| IBIS file stm32u575_585_wlcsp90_smps.ibs
[IBIS ver] 4.2
[File name] stm32u575_585_wlcsp90_smps.ibs
[File Rev] 1.0
[Date]  06-08-2021
[Source] Data Created at STMicroelectronics
[Notes]  File originated from ELDO simulations.
[Disclaimer]  This information is for modeling purpose only and is
   not guaranted. The information is subject to change without
   notice.
[Copyright] Copyright 2021 STMicroelectronics Inc.
|   Component stm32u575_585_wlcsp90_smps
[Component] stm32u575_585_wlcsp90_smps
[Manufacturer] STMicroelectronics
[Package]
| variable   typ   min   max
R_pkg   0   NA   NA
L_pkg   0   NA   NA
C_pkg   0   NA   NA
[Pin]   signal_name   model_name   R_pin   L_pin   C_pin   | Comment
A1 VDD POWER
A11 VDDIO2 POWER
A13 PB6 io8_100m_i2c_ft
A15 PB9 io8_100m_i2c_ft
A17 VDD11 POWER
A3 PC11 io8_100m_hslv_ft
A5 PD2 io8_100m_ft
A7 PG10 io8_100m_hslv_ft
A9 PG14 io8_100m_hslv_ft
B10 VSS GND
B12 PB7 io8_166m_hslv_i2c_ft
B14 PB8 io8_100m_i2c_ft
B16 VSS GND
B18 VDD POWER
B2 VSS GND
B4 PC12 io8_166m_hslv_ft
B6 PD5 io8_100m_hslv_ft
B8 PG12 io8_100m_hslv_ft
C1 VDDUSB POWER
C11 PB4 io8_100m_i2c_ft
C13 PH3-BOOT0 io8_100m_ft
C15 PE3 io8_100m_hslv_tamp_ft
C17 VBAT POWER
C3 PA14 io8_100m_ft
C5 PD0 io8_100m_hslv_ft
C7 PG9 io8_100m_hslv_ft
C9 PG13 io8_100m_hslv_ft
D10 PB3 io8_100m_i2c_ft
D12 PB5 io8_166m_hslv_ft
D14 PE4 io8_100m_hslv_tamp_ft
D16 PE6 io8_100m_hslv_tamp_ft
D18 PC14-OSC32_IN io8_100m_ft
D2 PA12 io8_usb_ft
D4 PA13 io8_100m_ft
D6 PD1 io8_100m_hslv_ft
D8 PD4 io8_100m_hslv_ft
E1 PA10 io8_100m_usb_id
E11 PA9 io8_100m_usb_vbus_ft
E13 PE5 io8_100m_hslv_tamp_ft
E15 PC13 io8_100m_ft_v33
E17 PC15-OSC32_OUT io8_100m_ft
E3 PA11 io8_usb_ft
E5 PA15 nc
E7 PC10 io8_100m_ft
E9 PG11 io8_100m_hslv_ft
F10 PA6 io8_100m_hslv_ft
F12 PC2 io8_100m_hslv_ft
F14 PC0 io8_100m_hslv_ft
F16 PH1-OSC_OUT io8_100m_ft
F18 PH0-OSC_IN io8_100m_ft
F2 PC8 io8_100m_ft
F4 PC7 io8_100m_ft
F6 PC9 io8_100m_ft
F8 PA8 io8_166m_hslv_ft
G1 PD14 io8_100m_hslv_ft
G11 PA0 io8_100m_hslv_tamp_ft
G13 PC3 io8_100m_hslv_ft
G15 PC1 io8_166m_hslv_i2c_ft
G17 NRST nc
G3 PD15 io8_100m_hslv_ft
G5 PB15 nc
G7 PC6 io8_100m_ft
G9 PC5 io8_100m_tamp_ft
H10 PA3 io8_166m_hslv_ft
H12 PA5 io8_100m_ft
H14 PA4 io8_100m_hslv_ft
H16 VREF+ POWER
H18 VSSA GND
H2 PB13 io8_100m_i2c_ft
H4 PB14 io8_100m_i2c_ft
H6 PB10 io8_166m_hslv_i2c_ft
H8 PE7 io8_100m_hslv_ft
J1 VDD POWER
J11 PB1 io8_100m_hslv_ft
J13 PA1 io8_100m_hslv_tamp_ft
J15 PA2 io8_100m_hslv_ft
J17 VDDA POWER
J3 VSS GND
J5 VSSSMPS GND
J7 PE10 io8_166m_hslv_ft
J9 PE8 io8_100m_hslv_ft
K10 PB2 io8_100m_hslv_tamp_ft
K12 PB0 io8_100m_hslv_ft
K14 PA7 io8_100m_hslv_ft
K16 VDD POWER
K18 VSS GND
K1 VDD11 POWER
K4 VDDSMPS POWER
K6 VLXSMPS POWER
K8 PE9 io8_166m_hslv_ft
[Model Selector] io8_100m_ft
io8_100m_ft_hs_1v2  "IO8_FT 100MHz high speed @ 1.2V"
io8_100m_ft_hs_pu_1v2  "IO8_FT 100MHz high speed @ 1.2V pullup"
io8_100m_ft_hs_pd_1v2  "IO8_FT 100MHz high speed @ 1.2V pulldown"
io8_100m_ft_fs_1v2  "IO8_FT 100MHz fast speed @ 1.2V"
io8_100m_ft_fs_pu_1v2  "IO8_FT 100MHz fast speed @ 1.2V pullup"
io8_100m_ft_fs_pd_1v2  "IO8_FT 100MHz fast speed @ 1.2V pulldown"
io8_100m_ft_ms_1v2  "IO8_FT 100MHz med speed @ 1.2V"
io8_100m_ft_ms_pu_1v2  "IO8_FT 100MHz med speed @ 1.2V pullup"
io8_100m_ft_ms_pd_1v2  "IO8_FT 100MHz med speed @ 1.2V pulldown"
io8_100m_ft_ls_1v2  "IO8_FT 100MHz low speed @ 1.2V"
io8_100m_ft_ls_pu_1v2  "IO8_FT 100MHz low speed @ 1.2V pullup"
io8_100m_ft_ls_pd_1v2  "IO8_FT 100MHz low speed @ 1.2V pulldown"
io8_100m_ft_hs_1v8  "IO8_FT 100MHz high speed @ 1.8V"
io8_100m_ft_hs_pu_1v8  "IO8_FT 100MHz high speed @ 1.8V pullup"
io8_100m_ft_hs_pd_1v8  "IO8_FT 100MHz high speed @ 1.8V pulldown"
io8_100m_ft_fs_1v8  "IO8_FT 100MHz fast speed @ 1.8V"
io8_100m_ft_fs_pu_1v8  "IO8_FT 100MHz fast speed @ 1.8V pullup"
io8_100m_ft_fs_pd_1v8  "IO8_FT 100MHz fast speed @ 1.8V pulldown"
io8_100m_ft_ms_1v8  "IO8_FT 100MHz med speed @ 1.8V"
io8_100m_ft_ms_pu_1v8  "IO8_FT 100MHz med speed @ 1.8V pullup"
io8_100m_ft_ms_pd_1v8  "IO8_FT 100MHz med speed @ 1.8V pulldown"
io8_100m_ft_ls_1v8  "IO8_FT 100MHz low speed @ 1.8V"
io8_100m_ft_ls_pu_1v8  "IO8_FT 100MHz low speed @ 1.8V pullup"
io8_100m_ft_ls_pd_1v8  "IO8_FT 100MHz low speed @ 1.8V pulldown"
io8_100m_ft_hs_3v3  "IO8_FT 100MHz high speed @ 3.3V"
io8_100m_ft_hs_pu_3v3  "IO8_FT 100MHz high speed @ 3.3V pullup"
io8_100m_ft_hs_pd_3v3  "IO8_FT 100MHz high speed @ 3.3V pulldown"
io8_100m_ft_fs_3v3  "IO8_FT 100MHz fast speed @ 3.3V"
io8_100m_ft_fs_pu_3v3  "IO8_FT 100MHz fast speed @ 3.3V pullup"
io8_100m_ft_fs_pd_3v3  "IO8_FT 100MHz fast speed @ 3.3V pulldown"
io8_100m_ft_ms_3v3  "IO8_FT 100MHz med speed @ 3.3V"
io8_100m_ft_ms_pu_3v3  "IO8_FT 100MHz med speed @ 3.3V pullup"
io8_100m_ft_ms_pd_3v3  "IO8_FT 100MHz med speed @ 3.3V pulldown"
io8_100m_ft_ls_3v3  "IO8_FT 100MHz low speed @ 3.3V"
io8_100m_ft_ls_pu_3v3  "IO8_FT 100MHz low speed @ 3.3V pullup"
io8_100m_ft_ls_pd_3v3  "IO8_FT 100MHz low speed @ 3.3V pulldown"
[Model Selector] io8_100m_hslv_ft
io8_100m_ft_hs_1v2  "IO8_FT 100MHz high speed @ 1.2V"
io8_100m_ft_hs_pu_1v2  "IO8_FT 100MHz high speed @ 1.2V pullup"
io8_100m_ft_hs_pd_1v2  "IO8_FT 100MHz high speed @ 1.2V pulldown"
io8_100m_ft_fs_1v2  "IO8_FT 100MHz fast speed @ 1.2V"
io8_100m_ft_fs_pu_1v2  "IO8_FT 100MHz fast speed @ 1.2V pullup"
io8_100m_ft_fs_pd_1v2  "IO8_FT 100MHz fast speed @ 1.2V pulldown"
io8_100m_ft_ms_1v2  "IO8_FT 100MHz med speed @ 1.2V"
io8_100m_ft_ms_pu_1v2  "IO8_FT 100MHz med speed @ 1.2V pullup"
io8_100m_ft_ms_pd_1v2  "IO8_FT 100MHz med speed @ 1.2V pulldown"
io8_100m_ft_ls_1v2  "IO8_FT 100MHz low speed @ 1.2V"
io8_100m_ft_ls_pu_1v2  "IO8_FT 100MHz low speed @ 1.2V pullup"
io8_100m_ft_ls_pd_1v2  "IO8_FT 100MHz low speed @ 1.2V pulldown"
io8_100m_ft_hs_1v8  "IO8_FT 100MHz high speed @ 1.8V"
io8_100m_ft_hs_pu_1v8  "IO8_FT 100MHz high speed @ 1.8V pullup"
io8_100m_ft_hs_pd_1v8  "IO8_FT 100MHz high speed @ 1.8V pulldown"
io8_100m_ft_fs_1v8  "IO8_FT 100MHz fast speed @ 1.8V"
io8_100m_ft_fs_pu_1v8  "IO8_FT 100MHz fast speed @ 1.8V pullup"
io8_100m_ft_fs_pd_1v8  "IO8_FT 100MHz fast speed @ 1.8V pulldown"
io8_100m_ft_ms_1v8  "IO8_FT 100MHz med speed @ 1.8V"
io8_100m_ft_ms_pu_1v8  "IO8_FT 100MHz med speed @ 1.8V pullup"
io8_100m_ft_ms_pd_1v8  "IO8_FT 100MHz med speed @ 1.8V pulldown"
io8_100m_ft_ls_1v8  "IO8_FT 100MHz low speed @ 1.8V"
io8_100m_ft_ls_pu_1v8  "IO8_FT 100MHz low speed @ 1.8V pullup"
io8_100m_ft_ls_pd_1v8  "IO8_FT 100MHz low speed @ 1.8V pulldown"
io8_100m_ft_hs_3v3  "IO8_FT 100MHz high speed @ 3.3V"
io8_100m_ft_hs_pu_3v3  "IO8_FT 100MHz high speed @ 3.3V pullup"
io8_100m_ft_hs_pd_3v3  "IO8_FT 100MHz high speed @ 3.3V pulldown"
io8_100m_ft_fs_3v3  "IO8_FT 100MHz fast speed @ 3.3V"
io8_100m_ft_fs_pu_3v3  "IO8_FT 100MHz fast speed @ 3.3V pullup"
io8_100m_ft_fs_pd_3v3  "IO8_FT 100MHz fast speed @ 3.3V pulldown"
io8_100m_ft_ms_3v3  "IO8_FT 100MHz med speed @ 3.3V"
io8_100m_ft_ms_pu_3v3  "IO8_FT 100MHz med speed @ 3.3V pullup"
io8_100m_ft_ms_pd_3v3  "IO8_FT 100MHz med speed @ 3.3V pulldown"
io8_100m_ft_ls_3v3  "IO8_FT 100MHz low speed @ 3.3V"
io8_100m_ft_ls_pu_3v3  "IO8_FT 100MHz low speed @ 3.3V pullup"
io8_100m_ft_ls_pd_3v3  "IO8_FT 100MHz low speed @ 3.3V pulldown"
io8_100m_hslv_ft_hs_1v2  "IO8_FT 100MHz HSLV high speed @ 1.2V"
io8_100m_hslv_ft_hs_pu_1v2  "IO8_FT 100MHz HSLV high speed @ 1.2V pullup"
io8_100m_hslv_ft_hs_pd_1v2  "IO8_FT 100MHz HSLV high speed @ 1.2V pulldown"
io8_100m_hslv_ft_fs_1v2  "IO8_FT 100MHz HSLV fast speed @ 1.2V"
io8_100m_hslv_ft_fs_pu_1v2  "IO8_FT 100MHz HSLV fast speed @ 1.2V pullup"
io8_100m_hslv_ft_fs_pd_1v2  "IO8_FT 100MHz HSLV fast speed @ 1.2V pulldown"
io8_100m_hslv_ft_ms_1v2  "IO8_FT 100MHz HSLV med speed @ 1.2V"
io8_100m_hslv_ft_ms_pu_1v2  "IO8_FT 100MHz HSLV med speed @ 1.2V pullup"
io8_100m_hslv_ft_ms_pd_1v2  "IO8_FT 100MHz HSLV med speed @ 1.2V pulldown"
io8_100m_hslv_ft_ls_1v2  "IO8_FT 100MHz HSLV low speed @ 1.2V"
io8_100m_hslv_ft_ls_pu_1v2  "IO8_FT 100MHz HSLV low speed @ 1.2V pullup"
io8_100m_hslv_ft_ls_pd_1v2  "IO8_FT 100MHz HSLV low speed @ 1.2V pulldown"
io8_100m_hslv_ft_hs_1v8  "IO8_FT 100MHz HSLV high speed @ 1.8V"
io8_100m_hslv_ft_hs_pu_1v8  "IO8_FT 100MHz HSLV high speed @ 1.8V pullup"
io8_100m_hslv_ft_hs_pd_1v8  "IO8_FT 100MHz HSLV high speed @ 1.8V pulldown"
io8_100m_hslv_ft_fs_1v8  "IO8_FT 100MHz HSLV fast speed @ 1.8V"
io8_100m_hslv_ft_fs_pu_1v8  "IO8_FT 100MHz HSLV fast speed @ 1.8V pullup"
io8_100m_hslv_ft_fs_pd_1v8  "IO8_FT 100MHz HSLV fast speed @ 1.8V pulldown"
io8_100m_hslv_ft_ms_1v8  "IO8_FT 100MHz HSLV med speed @ 1.8V"
io8_100m_hslv_ft_ms_pu_1v8  "IO8_FT 100MHz HSLV med speed @ 1.8V pullup"
io8_100m_hslv_ft_ms_pd_1v8  "IO8_FT 100MHz HSLV med speed @ 1.8V pulldown"
io8_100m_hslv_ft_ls_1v8  "IO8_FT 100MHz HSLV low speed @ 1.8V"
io8_100m_hslv_ft_ls_pu_1v8  "IO8_FT 100MHz HSLV low speed @ 1.8V pullup"
io8_100m_hslv_ft_ls_pd_1v8  "IO8_FT 100MHz HSLV low speed @ 1.8V pulldown"
io8_100m_hslv_ft_hs_2v5  "IO8_FT 100MHz HSLV high speed @ 2.5V"
io8_100m_hslv_ft_hs_pu_2v5  "IO8_FT 100MHz HSLV high speed @ 2.5V pullup"
io8_100m_hslv_ft_hs_pd_2v5  "IO8_FT 100MHz HSLV high speed @ 2.5V pulldown"
io8_100m_hslv_ft_fs_2v5  "IO8_FT 100MHz HSLV fast speed @ 2.5V"
io8_100m_hslv_ft_fs_pu_2v5  "IO8_FT 100MHz HSLV fast speed @ 2.5V pullup"
io8_100m_hslv_ft_fs_pd_2v5  "IO8_FT 100MHz HSLV fast speed @ 2.5V pulldown"
io8_100m_hslv_ft_ms_2v5  "IO8_FT 100MHz HSLV med speed @ 2.5V"
io8_100m_hslv_ft_ms_pu_2v5  "IO8_FT 100MHz HSLV med speed @ 2.5V pullup"
io8_100m_hslv_ft_ms_pd_2v5  "IO8_FT 100MHz HSLV med speed @ 2.5V pulldown"
io8_100m_hslv_ft_ls_2v5  "IO8_FT 100MHz HSLV low speed @ 2.5V"
io8_100m_hslv_ft_ls_pu_2v5  "IO8_FT 100MHz HSLV low speed @ 2.5V pullup"
io8_100m_hslv_ft_ls_pd_2v5  "IO8_FT 100MHz HSLV low speed @ 2.5V pulldown"
[Model Selector] io8_166m_hslv_ft
io8_166m_ft_hs_1v2  "IO8_FT 166MHz high speed @ 1.2V"
io8_166m_ft_hs_pu_1v2  "IO8_FT 166MHz high speed @ 1.2V pullup"
io8_166m_ft_hs_pd_1v2  "IO8_FT 166MHz high speed @ 1.2V pulldown"
io8_166m_ft_fs_1v2  "IO8_FT 166MHz fast speed @ 1.2V"
io8_166m_ft_fs_pu_1v2  "IO8_FT 166MHz fast speed @ 1.2V pullup"
io8_166m_ft_fs_pd_1v2  "IO8_FT 166MHz fast speed @ 1.2V pulldown"
io8_166m_ft_ms_1v2  "IO8_FT 166MHz med speed @ 1.2V"
io8_166m_ft_ms_pu_1v2  "IO8_FT 166MHz med speed @ 1.2V pullup"
io8_166m_ft_ms_pd_1v2  "IO8_FT 166MHz med speed @ 1.2V pulldown"
io8_166m_ft_ls_1v2  "IO8_FT 166MHz low speed @ 1.2V"
io8_166m_ft_ls_pu_1v2  "IO8_FT 166MHz low speed @ 1.2V pullup"
io8_166m_ft_ls_pd_1v2  "IO8_FT 166MHz low speed @ 1.2V pulldown"
io8_166m_ft_hs_1v8  "IO8_FT 166MHz high speed @ 1.8V"
io8_166m_ft_hs_pu_1v8  "IO8_FT 166MHz high speed @ 1.8V pullup"
io8_166m_ft_hs_pd_1v8  "IO8_FT 166MHz high speed @ 1.8V pulldown"
io8_166m_ft_fs_1v8  "IO8_FT 166MHz fast speed @ 1.8V"
io8_166m_ft_fs_pu_1v8  "IO8_FT 166MHz fast speed @ 1.8V pullup"
io8_166m_ft_fs_pd_1v8  "IO8_FT 166MHz fast speed @ 1.8V pulldown"
io8_166m_ft_ms_1v8  "IO8_FT 166MHz med speed @ 1.8V"
io8_166m_ft_ms_pu_1v8  "IO8_FT 166MHz med speed @ 1.8V pullup"
io8_166m_ft_ms_pd_1v8  "IO8_FT 166MHz med speed @ 1.8V pulldown"
io8_166m_ft_ls_1v8  "IO8_FT 166MHz low speed @ 1.8V"
io8_166m_ft_ls_pu_1v8  "IO8_FT 166MHz low speed @ 1.8V pullup"
io8_166m_ft_ls_pd_1v8  "IO8_FT 166MHz low speed @ 1.8V pulldown"
io8_166m_ft_hs_3v3  "IO8_FT 166MHz high speed @ 3.3V"
io8_166m_ft_hs_pu_3v3  "IO8_FT 166MHz high speed @ 3.3V pullup"
io8_166m_ft_hs_pd_3v3  "IO8_FT 166MHz high speed @ 3.3V pulldown"
io8_166m_ft_fs_3v3  "IO8_FT 166MHz fast speed @ 3.3V"
io8_166m_ft_fs_pu_3v3  "IO8_FT 166MHz fast speed @ 3.3V pullup"
io8_166m_ft_fs_pd_3v3  "IO8_FT 166MHz fast speed @ 3.3V pulldown"
io8_166m_ft_ms_3v3  "IO8_FT 166MHz med speed @ 3.3V"
io8_166m_ft_ms_pu_3v3  "IO8_FT 166MHz med speed @ 3.3V pullup"
io8_166m_ft_ms_pd_3v3  "IO8_FT 166MHz med speed @ 3.3V pulldown"
io8_166m_ft_ls_3v3  "IO8_FT 166MHz low speed @ 3.3V"
io8_166m_ft_ls_pu_3v3  "IO8_FT 166MHz low speed @ 3.3V pullup"
io8_166m_ft_ls_pd_3v3  "IO8_FT 166MHz low speed @ 3.3V pulldown"
io8_166m_hslv_ft_hs_1v2  "IO8_FT 166MHz HSLV high speed @ 1.2V"
io8_166m_hslv_ft_hs_pu_1v2  "IO8_FT 166MHz HSLV high speed @ 1.2V pullup"
io8_166m_hslv_ft_hs_pd_1v2  "IO8_FT 166MHz HSLV high speed @ 1.2V pulldown"
io8_166m_hslv_ft_fs_1v2  "IO8_FT 166MHz HSLV fast speed @ 1.2V"
io8_166m_hslv_ft_fs_pu_1v2  "IO8_FT 166MHz HSLV fast speed @ 1.2V pullup"
io8_166m_hslv_ft_fs_pd_1v2  "IO8_FT 166MHz HSLV fast speed @ 1.2V pulldown"
io8_166m_hslv_ft_ms_1v2  "IO8_FT 166MHz HSLV med speed @ 1.2V"
io8_166m_hslv_ft_ms_pu_1v2  "IO8_FT 166MHz HSLV med speed @ 1.2V pullup"
io8_166m_hslv_ft_ms_pd_1v2  "IO8_FT 166MHz HSLV med speed @ 1.2V pulldown"
io8_166m_hslv_ft_ls_1v2  "IO8_FT 166MHz HSLV low speed @ 1.2V"
io8_166m_hslv_ft_ls_pu_1v2  "IO8_FT 166MHz HSLV low speed @ 1.2V pullup"
io8_166m_hslv_ft_ls_pd_1v2  "IO8_FT 166MHz HSLV low speed @ 1.2V pulldown"
io8_166m_hslv_ft_hs_1v8  "IO8_FT 166MHz HSLV high speed @ 1.8V"
io8_166m_hslv_ft_hs_pu_1v8  "IO8_FT 166MHz HSLV high speed @ 1.8V pullup"
io8_166m_hslv_ft_hs_pd_1v8  "IO8_FT 166MHz HSLV high speed @ 1.8V pulldown"
io8_166m_hslv_ft_fs_1v8  "IO8_FT 166MHz HSLV fast speed @ 1.8V"
io8_166m_hslv_ft_fs_pu_1v8  "IO8_FT 166MHz HSLV fast speed @ 1.8V pullup"
io8_166m_hslv_ft_fs_pd_1v8  "IO8_FT 166MHz HSLV fast speed @ 1.8V pulldown"
io8_166m_hslv_ft_ms_1v8  "IO8_FT 166MHz HSLV med speed @ 1.8V"
io8_166m_hslv_ft_ms_pu_1v8  "IO8_FT 166MHz HSLV med speed @ 1.8V pullup"
io8_166m_hslv_ft_ms_pd_1v8  "IO8_FT 166MHz HSLV med speed @ 1.8V pulldown"
io8_166m_hslv_ft_ls_1v8  "IO8_FT 166MHz HSLV low speed @ 1.8V"
io8_166m_hslv_ft_ls_pu_1v8  "IO8_FT 166MHz HSLV low speed @ 1.8V pullup"
io8_166m_hslv_ft_ls_pd_1v8  "IO8_FT 166MHz HSLV low speed @ 1.8V pulldown"
io8_166m_hslv_ft_hs_2v5  "IO8_FT 166MHz HSLV high speed @ 2.5V"
io8_166m_hslv_ft_hs_pu_2v5  "IO8_FT 166MHz HSLV high speed @ 2.5V pullup"
io8_166m_hslv_ft_hs_pd_2v5  "IO8_FT 166MHz HSLV high speed @ 2.5V pulldown"
io8_166m_hslv_ft_fs_2v5  "IO8_FT 166MHz HSLV fast speed @ 2.5V"
io8_166m_hslv_ft_fs_pu_2v5  "IO8_FT 166MHz HSLV fast speed @ 2.5V pullup"
io8_166m_hslv_ft_fs_pd_2v5  "IO8_FT 166MHz HSLV fast speed @ 2.5V pulldown"
io8_166m_hslv_ft_ms_2v5  "IO8_FT 166MHz HSLV med speed @ 2.5V"
io8_166m_hslv_ft_ms_pu_2v5  "IO8_FT 166MHz HSLV med speed @ 2.5V pullup"
io8_166m_hslv_ft_ms_pd_2v5  "IO8_FT 166MHz HSLV med speed @ 2.5V pulldown"
io8_166m_hslv_ft_ls_2v5  "IO8_FT 166MHz HSLV low speed @ 2.5V"
io8_166m_hslv_ft_ls_pu_2v5  "IO8_FT 166MHz HSLV low speed @ 2.5V pullup"
io8_166m_hslv_ft_ls_pd_2v5  "IO8_FT 166MHz HSLV low speed @ 2.5V pulldown"
[Model Selector] io8_100m_ft_v33
io8_ft_v33_hs_1v2  "IO8_FT_V33 high speed @ 1.2V"
io8_ft_v33_hs_pu_1v2  "IO8_FT_V33 high speed @ 1.2V pullup"
io8_ft_v33_hs_pd_1v2  "IO8_FT_V33 high speed @ 1.2V pulldown"
io8_ft_v33_fs_1v2  "IO8_FT_V33 fast speed @ 1.2V"
io8_ft_v33_fs_pu_1v2  "IO8_FT_V33 fast speed @ 1.2V pullup"
io8_ft_v33_fs_pd_1v2  "IO8_FT_V33 fast speed @ 1.2V pulldown"
io8_ft_v33_ms_1v2  "IO8_FT_V33 med speed @ 1.2V"
io8_ft_v33_ms_pu_1v2  "IO8_FT_V33 med speed @ 1.2V pullup"
io8_ft_v33_ms_pd_1v2  "IO8_FT_V33 med speed @ 1.2V pulldown"
io8_ft_v33_ls_1v2  "IO8_FT_V33 low speed @ 1.2V"
io8_ft_v33_ls_pu_1v2  "IO8_FT_V33 low speed @ 1.2V pullup"
io8_ft_v33_ls_pd_1v2  "IO8_FT_V33 low speed @ 1.2V pulldown"
io8_ft_v33_hs_1v8  "IO8_FT_V33 high speed @ 1.8V"
io8_ft_v33_hs_pu_1v8  "IO8_FT_V33 high speed @ 1.8V pullup"
io8_ft_v33_hs_pd_1v8  "IO8_FT_V33 high speed @ 1.8V pulldown"
io8_ft_v33_fs_1v8  "IO8_FT_V33 fast speed @ 1.8V"
io8_ft_v33_fs_pu_1v8  "IO8_FT_V33 fast speed @ 1.8V pullup"
io8_ft_v33_fs_pd_1v8  "IO8_FT_V33 fast speed @ 1.8V pulldown"
io8_ft_v33_ms_1v8  "IO8_FT_V33 med speed @ 1.8V"
io8_ft_v33_ms_pu_1v8  "IO8_FT_V33 med speed @ 1.8V pullup"
io8_ft_v33_ms_pd_1v8  "IO8_FT_V33 med speed @ 1.8V pulldown"
io8_ft_v33_ls_1v8  "IO8_FT_V33 low speed @ 1.8V"
io8_ft_v33_ls_pu_1v8  "IO8_FT_V33 low speed @ 1.8V pullup"
io8_ft_v33_ls_pd_1v8  "IO8_FT_V33 low speed @ 1.8V pulldown"
io8_ft_v33_hs_3v3  "IO8_FT_V33 high speed @ 3.3V"
io8_ft_v33_hs_pu_3v3  "IO8_FT_V33 high speed @ 3.3V pullup"
io8_ft_v33_hs_pd_3v3  "IO8_FT_V33 high speed @ 3.3V pulldown"
io8_ft_v33_fs_3v3  "IO8_FT_V33 fast speed @ 3.3V"
io8_ft_v33_fs_pu_3v3  "IO8_FT_V33 fast speed @ 3.3V pullup"
io8_ft_v33_fs_pd_3v3  "IO8_FT_V33 fast speed @ 3.3V pulldown"
io8_ft_v33_ms_3v3  "IO8_FT_V33 med speed @ 3.3V"
io8_ft_v33_ms_pu_3v3  "IO8_FT_V33 med speed @ 3.3V pullup"
io8_ft_v33_ms_pd_3v3  "IO8_FT_V33 med speed @ 3.3V pulldown"
io8_ft_v33_ls_3v3  "IO8_FT_V33 low speed @ 3.3V"
io8_ft_v33_ls_pu_3v3  "IO8_FT_V33 low speed @ 3.3V pullup"
io8_ft_v33_ls_pd_3v3  "IO8_FT_V33 low speed @ 3.3V pulldown"
[Model Selector] io8_100m_tamp_ft
io8_100m_ft_hs_1v2  "IO8_FT 100MHz high speed @ 1.2V"
io8_100m_ft_hs_pu_1v2  "IO8_FT 100MHz high speed @ 1.2V pullup"
io8_100m_ft_hs_pd_1v2  "IO8_FT 100MHz high speed @ 1.2V pulldown"
io8_100m_ft_fs_1v2  "IO8_FT 100MHz fast speed @ 1.2V"
io8_100m_ft_fs_pu_1v2  "IO8_FT 100MHz fast speed @ 1.2V pullup"
io8_100m_ft_fs_pd_1v2  "IO8_FT 100MHz fast speed @ 1.2V pulldown"
io8_100m_ft_ms_1v2  "IO8_FT 100MHz med speed @ 1.2V"
io8_100m_ft_ms_pu_1v2  "IO8_FT 100MHz med speed @ 1.2V pullup"
io8_100m_ft_ms_pd_1v2  "IO8_FT 100MHz med speed @ 1.2V pulldown"
io8_100m_ft_ls_1v2  "IO8_FT 100MHz low speed @ 1.2V"
io8_100m_ft_ls_pu_1v2  "IO8_FT 100MHz low speed @ 1.2V pullup"
io8_100m_ft_ls_pd_1v2  "IO8_FT 100MHz low speed @ 1.2V pulldown"
io8_100m_ft_hs_1v8  "IO8_FT 100MHz high speed @ 1.8V"
io8_100m_ft_hs_pu_1v8  "IO8_FT 100MHz high speed @ 1.8V pullup"
io8_100m_ft_hs_pd_1v8  "IO8_FT 100MHz high speed @ 1.8V pulldown"
io8_100m_ft_fs_1v8  "IO8_FT 100MHz fast speed @ 1.8V"
io8_100m_ft_fs_pu_1v8  "IO8_FT 100MHz fast speed @ 1.8V pullup"
io8_100m_ft_fs_pd_1v8  "IO8_FT 100MHz fast speed @ 1.8V pulldown"
io8_100m_ft_ms_1v8  "IO8_FT 100MHz med speed @ 1.8V"
io8_100m_ft_ms_pu_1v8  "IO8_FT 100MHz med speed @ 1.8V pullup"
io8_100m_ft_ms_pd_1v8  "IO8_FT 100MHz med speed @ 1.8V pulldown"
io8_100m_ft_ls_1v8  "IO8_FT 100MHz low speed @ 1.8V"
io8_100m_ft_ls_pu_1v8  "IO8_FT 100MHz low speed @ 1.8V pullup"
io8_100m_ft_ls_pd_1v8  "IO8_FT 100MHz low speed @ 1.8V pulldown"
io8_100m_ft_hs_3v3  "IO8_FT 100MHz high speed @ 3.3V"
io8_100m_ft_hs_pu_3v3  "IO8_FT 100MHz high speed @ 3.3V pullup"
io8_100m_ft_hs_pd_3v3  "IO8_FT 100MHz high speed @ 3.3V pulldown"
io8_100m_ft_fs_3v3  "IO8_FT 100MHz fast speed @ 3.3V"
io8_100m_ft_fs_pu_3v3  "IO8_FT 100MHz fast speed @ 3.3V pullup"
io8_100m_ft_fs_pd_3v3  "IO8_FT 100MHz fast speed @ 3.3V pulldown"
io8_100m_ft_ms_3v3  "IO8_FT 100MHz med speed @ 3.3V"
io8_100m_ft_ms_pu_3v3  "IO8_FT 100MHz med speed @ 3.3V pullup"
io8_100m_ft_ms_pd_3v3  "IO8_FT 100MHz med speed @ 3.3V pulldown"
io8_100m_ft_ls_3v3  "IO8_FT 100MHz low speed @ 3.3V"
io8_100m_ft_ls_pu_3v3  "IO8_FT 100MHz low speed @ 3.3V pullup"
io8_100m_ft_ls_pd_3v3  "IO8_FT 100MHz low speed @ 3.3V pulldown"
io8_ft_v33_hs_1v2  "IO8_FT_V33 high speed @ 1.2V"
io8_ft_v33_hs_pu_1v2  "IO8_FT_V33 high speed @ 1.2V pullup"
io8_ft_v33_hs_pd_1v2  "IO8_FT_V33 high speed @ 1.2V pulldown"
io8_ft_v33_fs_1v2  "IO8_FT_V33 fast speed @ 1.2V"
io8_ft_v33_fs_pu_1v2  "IO8_FT_V33 fast speed @ 1.2V pullup"
io8_ft_v33_fs_pd_1v2  "IO8_FT_V33 fast speed @ 1.2V pulldown"
io8_ft_v33_ms_1v2  "IO8_FT_V33 med speed @ 1.2V"
io8_ft_v33_ms_pu_1v2  "IO8_FT_V33 med speed @ 1.2V pullup"
io8_ft_v33_ms_pd_1v2  "IO8_FT_V33 med speed @ 1.2V pulldown"
io8_ft_v33_ls_1v2  "IO8_FT_V33 low speed @ 1.2V"
io8_ft_v33_ls_pu_1v2  "IO8_FT_V33 low speed @ 1.2V pullup"
io8_ft_v33_ls_pd_1v2  "IO8_FT_V33 low speed @ 1.2V pulldown"
io8_ft_v33_hs_1v8  "IO8_FT_V33 high speed @ 1.8V"
io8_ft_v33_hs_pu_1v8  "IO8_FT_V33 high speed @ 1.8V pullup"
io8_ft_v33_hs_pd_1v8  "IO8_FT_V33 high speed @ 1.8V pulldown"
io8_ft_v33_fs_1v8  "IO8_FT_V33 fast speed @ 1.8V"
io8_ft_v33_fs_pu_1v8  "IO8_FT_V33 fast speed @ 1.8V pullup"
io8_ft_v33_fs_pd_1v8  "IO8_FT_V33 fast speed @ 1.8V pulldown"
io8_ft_v33_ms_1v8  "IO8_FT_V33 med speed @ 1.8V"
io8_ft_v33_ms_pu_1v8  "IO8_FT_V33 med speed @ 1.8V pullup"
io8_ft_v33_ms_pd_1v8  "IO8_FT_V33 med speed @ 1.8V pulldown"
io8_ft_v33_ls_1v8  "IO8_FT_V33 low speed @ 1.8V"
io8_ft_v33_ls_pu_1v8  "IO8_FT_V33 low speed @ 1.8V pullup"
io8_ft_v33_ls_pd_1v8  "IO8_FT_V33 low speed @ 1.8V pulldown"
io8_ft_v33_hs_3v3  "IO8_FT_V33 high speed @ 3.3V"
io8_ft_v33_hs_pu_3v3  "IO8_FT_V33 high speed @ 3.3V pullup"
io8_ft_v33_hs_pd_3v3  "IO8_FT_V33 high speed @ 3.3V pulldown"
io8_ft_v33_fs_3v3  "IO8_FT_V33 fast speed @ 3.3V"
io8_ft_v33_fs_pu_3v3  "IO8_FT_V33 fast speed @ 3.3V pullup"
io8_ft_v33_fs_pd_3v3  "IO8_FT_V33 fast speed @ 3.3V pulldown"
io8_ft_v33_ms_3v3  "IO8_FT_V33 med speed @ 3.3V"
io8_ft_v33_ms_pu_3v3  "IO8_FT_V33 med speed @ 3.3V pullup"
io8_ft_v33_ms_pd_3v3  "IO8_FT_V33 med speed @ 3.3V pulldown"
io8_ft_v33_ls_3v3  "IO8_FT_V33 low speed @ 3.3V"
io8_ft_v33_ls_pu_3v3  "IO8_FT_V33 low speed @ 3.3V pullup"
io8_ft_v33_ls_pd_3v3  "IO8_FT_V33 low speed @ 3.3V pulldown"
[Model Selector] io8_100m_hslv_tamp_ft
io8_100m_ft_hs_1v2  "IO8_FT 100MHz high speed @ 1.2V"
io8_100m_ft_hs_pu_1v2  "IO8_FT 100MHz high speed @ 1.2V pullup"
io8_100m_ft_hs_pd_1v2  "IO8_FT 100MHz high speed @ 1.2V pulldown"
io8_100m_ft_fs_1v2  "IO8_FT 100MHz fast speed @ 1.2V"
io8_100m_ft_fs_pu_1v2  "IO8_FT 100MHz fast speed @ 1.2V pullup"
io8_100m_ft_fs_pd_1v2  "IO8_FT 100MHz fast speed @ 1.2V pulldown"
io8_100m_ft_ms_1v2  "IO8_FT 100MHz med speed @ 1.2V"
io8_100m_ft_ms_pu_1v2  "IO8_FT 100MHz med speed @ 1.2V pullup"
io8_100m_ft_ms_pd_1v2  "IO8_FT 100MHz med speed @ 1.2V pulldown"
io8_100m_ft_ls_1v2  "IO8_FT 100MHz low speed @ 1.2V"
io8_100m_ft_ls_pu_1v2  "IO8_FT 100MHz low speed @ 1.2V pullup"
io8_100m_ft_ls_pd_1v2  "IO8_FT 100MHz low speed @ 1.2V pulldown"
io8_100m_ft_hs_1v8  "IO8_FT 100MHz high speed @ 1.8V"
io8_100m_ft_hs_pu_1v8  "IO8_FT 100MHz high speed @ 1.8V pullup"
io8_100m_ft_hs_pd_1v8  "IO8_FT 100MHz high speed @ 1.8V pulldown"
io8_100m_ft_fs_1v8  "IO8_FT 100MHz fast speed @ 1.8V"
io8_100m_ft_fs_pu_1v8  "IO8_FT 100MHz fast speed @ 1.8V pullup"
io8_100m_ft_fs_pd_1v8  "IO8_FT 100MHz fast speed @ 1.8V pulldown"
io8_100m_ft_ms_1v8  "IO8_FT 100MHz med speed @ 1.8V"
io8_100m_ft_ms_pu_1v8  "IO8_FT 100MHz med speed @ 1.8V pullup"
io8_100m_ft_ms_pd_1v8  "IO8_FT 100MHz med speed @ 1.8V pulldown"
io8_100m_ft_ls_1v8  "IO8_FT 100MHz low speed @ 1.8V"
io8_100m_ft_ls_pu_1v8  "IO8_FT 100MHz low speed @ 1.8V pullup"
io8_100m_ft_ls_pd_1v8  "IO8_FT 100MHz low speed @ 1.8V pulldown"
io8_100m_ft_hs_3v3  "IO8_FT 100MHz high speed @ 3.3V"
io8_100m_ft_hs_pu_3v3  "IO8_FT 100MHz high speed @ 3.3V pullup"
io8_100m_ft_hs_pd_3v3  "IO8_FT 100MHz high speed @ 3.3V pulldown"
io8_100m_ft_fs_3v3  "IO8_FT 100MHz fast speed @ 3.3V"
io8_100m_ft_fs_pu_3v3  "IO8_FT 100MHz fast speed @ 3.3V pullup"
io8_100m_ft_fs_pd_3v3  "IO8_FT 100MHz fast speed @ 3.3V pulldown"
io8_100m_ft_ms_3v3  "IO8_FT 100MHz med speed @ 3.3V"
io8_100m_ft_ms_pu_3v3  "IO8_FT 100MHz med speed @ 3.3V pullup"
io8_100m_ft_ms_pd_3v3  "IO8_FT 100MHz med speed @ 3.3V pulldown"
io8_100m_ft_ls_3v3  "IO8_FT 100MHz low speed @ 3.3V"
io8_100m_ft_ls_pu_3v3  "IO8_FT 100MHz low speed @ 3.3V pullup"
io8_100m_ft_ls_pd_3v3  "IO8_FT 100MHz low speed @ 3.3V pulldown"
io8_100m_hslv_ft_hs_1v2  "IO8_FT 100MHz HSLV high speed @ 1.2V"
io8_100m_hslv_ft_hs_pu_1v2  "IO8_FT 100MHz HSLV high speed @ 1.2V pullup"
io8_100m_hslv_ft_hs_pd_1v2  "IO8_FT 100MHz HSLV high speed @ 1.2V pulldown"
io8_100m_hslv_ft_fs_1v2  "IO8_FT 100MHz HSLV fast speed @ 1.2V"
io8_100m_hslv_ft_fs_pu_1v2  "IO8_FT 100MHz HSLV fast speed @ 1.2V pullup"
io8_100m_hslv_ft_fs_pd_1v2  "IO8_FT 100MHz HSLV fast speed @ 1.2V pulldown"
io8_100m_hslv_ft_ms_1v2  "IO8_FT 100MHz HSLV med speed @ 1.2V"
io8_100m_hslv_ft_ms_pu_1v2  "IO8_FT 100MHz HSLV med speed @ 1.2V pullup"
io8_100m_hslv_ft_ms_pd_1v2  "IO8_FT 100MHz HSLV med speed @ 1.2V pulldown"
io8_100m_hslv_ft_ls_1v2  "IO8_FT 100MHz HSLV low speed @ 1.2V"
io8_100m_hslv_ft_ls_pu_1v2  "IO8_FT 100MHz HSLV low speed @ 1.2V pullup"
io8_100m_hslv_ft_ls_pd_1v2  "IO8_FT 100MHz HSLV low speed @ 1.2V pulldown"
io8_100m_hslv_ft_hs_1v8  "IO8_FT 100MHz HSLV high speed @ 1.8V"
io8_100m_hslv_ft_hs_pu_1v8  "IO8_FT 100MHz HSLV high speed @ 1.8V pullup"
io8_100m_hslv_ft_hs_pd_1v8  "IO8_FT 100MHz HSLV high speed @ 1.8V pulldown"
io8_100m_hslv_ft_fs_1v8  "IO8_FT 100MHz HSLV fast speed @ 1.8V"
io8_100m_hslv_ft_fs_pu_1v8  "IO8_FT 100MHz HSLV fast speed @ 1.8V pullup"
io8_100m_hslv_ft_fs_pd_1v8  "IO8_FT 100MHz HSLV fast speed @ 1.8V pulldown"
io8_100m_hslv_ft_ms_1v8  "IO8_FT 100MHz HSLV med speed @ 1.8V"
io8_100m_hslv_ft_ms_pu_1v8  "IO8_FT 100MHz HSLV med speed @ 1.8V pullup"
io8_100m_hslv_ft_ms_pd_1v8  "IO8_FT 100MHz HSLV med speed @ 1.8V pulldown"
io8_100m_hslv_ft_ls_1v8  "IO8_FT 100MHz HSLV low speed @ 1.8V"
io8_100m_hslv_ft_ls_pu_1v8  "IO8_FT 100MHz HSLV low speed @ 1.8V pullup"
io8_100m_hslv_ft_ls_pd_1v8  "IO8_FT 100MHz HSLV low speed @ 1.8V pulldown"
io8_100m_hslv_ft_hs_2v5  "IO8_FT 100MHz HSLV high speed @ 2.5V"
io8_100m_hslv_ft_hs_pu_2v5  "IO8_FT 100MHz HSLV high speed @ 2.5V pullup"
io8_100m_hslv_ft_hs_pd_2v5  "IO8_FT 100MHz HSLV high speed @ 2.5V pulldown"
io8_100m_hslv_ft_fs_2v5  "IO8_FT 100MHz HSLV fast speed @ 2.5V"
io8_100m_hslv_ft_fs_pu_2v5  "IO8_FT 100MHz HSLV fast speed @ 2.5V pullup"
io8_100m_hslv_ft_fs_pd_2v5  "IO8_FT 100MHz HSLV fast speed @ 2.5V pulldown"
io8_100m_hslv_ft_ms_2v5  "IO8_FT 100MHz HSLV med speed @ 2.5V"
io8_100m_hslv_ft_ms_pu_2v5  "IO8_FT 100MHz HSLV med speed @ 2.5V pullup"
io8_100m_hslv_ft_ms_pd_2v5  "IO8_FT 100MHz HSLV med speed @ 2.5V pulldown"
io8_100m_hslv_ft_ls_2v5  "IO8_FT 100MHz HSLV low speed @ 2.5V"
io8_100m_hslv_ft_ls_pu_2v5  "IO8_FT 100MHz HSLV low speed @ 2.5V pullup"
io8_100m_hslv_ft_ls_pd_2v5  "IO8_FT 100MHz HSLV low speed @ 2.5V pulldown"
io8_ft_v33_hs_1v2  "IO8_FT_V33 high speed @ 1.2V"
io8_ft_v33_hs_pu_1v2  "IO8_FT_V33 high speed @ 1.2V pullup"
io8_ft_v33_hs_pd_1v2  "IO8_FT_V33 high speed @ 1.2V pulldown"
io8_ft_v33_fs_1v2  "IO8_FT_V33 fast speed @ 1.2V"
io8_ft_v33_fs_pu_1v2  "IO8_FT_V33 fast speed @ 1.2V pullup"
io8_ft_v33_fs_pd_1v2  "IO8_FT_V33 fast speed @ 1.2V pulldown"
io8_ft_v33_ms_1v2  "IO8_FT_V33 med speed @ 1.2V"
io8_ft_v33_ms_pu_1v2  "IO8_FT_V33 med speed @ 1.2V pullup"
io8_ft_v33_ms_pd_1v2  "IO8_FT_V33 med speed @ 1.2V pulldown"
io8_ft_v33_ls_1v2  "IO8_FT_V33 low speed @ 1.2V"
io8_ft_v33_ls_pu_1v2  "IO8_FT_V33 low speed @ 1.2V pullup"
io8_ft_v33_ls_pd_1v2  "IO8_FT_V33 low speed @ 1.2V pulldown"
io8_ft_v33_hs_1v8  "IO8_FT_V33 high speed @ 1.8V"
io8_ft_v33_hs_pu_1v8  "IO8_FT_V33 high speed @ 1.8V pullup"
io8_ft_v33_hs_pd_1v8  "IO8_FT_V33 high speed @ 1.8V pulldown"
io8_ft_v33_fs_1v8  "IO8_FT_V33 fast speed @ 1.8V"
io8_ft_v33_fs_pu_1v8  "IO8_FT_V33 fast speed @ 1.8V pullup"
io8_ft_v33_fs_pd_1v8  "IO8_FT_V33 fast speed @ 1.8V pulldown"
io8_ft_v33_ms_1v8  "IO8_FT_V33 med speed @ 1.8V"
io8_ft_v33_ms_pu_1v8  "IO8_FT_V33 med speed @ 1.8V pullup"
io8_ft_v33_ms_pd_1v8  "IO8_FT_V33 med speed @ 1.8V pulldown"
io8_ft_v33_ls_1v8  "IO8_FT_V33 low speed @ 1.8V"
io8_ft_v33_ls_pu_1v8  "IO8_FT_V33 low speed @ 1.8V pullup"
io8_ft_v33_ls_pd_1v8  "IO8_FT_V33 low speed @ 1.8V pulldown"
io8_ft_v33_hs_3v3  "IO8_FT_V33 high speed @ 3.3V"
io8_ft_v33_hs_pu_3v3  "IO8_FT_V33 high speed @ 3.3V pullup"
io8_ft_v33_hs_pd_3v3  "IO8_FT_V33 high speed @ 3.3V pulldown"
io8_ft_v33_fs_3v3  "IO8_FT_V33 fast speed @ 3.3V"
io8_ft_v33_fs_pu_3v3  "IO8_FT_V33 fast speed @ 3.3V pullup"
io8_ft_v33_fs_pd_3v3  "IO8_FT_V33 fast speed @ 3.3V pulldown"
io8_ft_v33_ms_3v3  "IO8_FT_V33 med speed @ 3.3V"
io8_ft_v33_ms_pu_3v3  "IO8_FT_V33 med speed @ 3.3V pullup"
io8_ft_v33_ms_pd_3v3  "IO8_FT_V33 med speed @ 3.3V pulldown"
io8_ft_v33_ls_3v3  "IO8_FT_V33 low speed @ 3.3V"
io8_ft_v33_ls_pu_3v3  "IO8_FT_V33 low speed @ 3.3V pullup"
io8_ft_v33_ls_pd_3v3  "IO8_FT_V33 low speed @ 3.3V pulldown"
[Model Selector] io8_100m_usb_id
io8_100m_ft_hs_1v2  "IO8_FT 100MHz high speed @ 1.2V"
io8_100m_ft_hs_pu_1v2  "IO8_FT 100MHz high speed @ 1.2V pullup"
io8_100m_ft_hs_pd_1v2  "IO8_FT 100MHz high speed @ 1.2V pulldown"
io8_100m_ft_fs_1v2  "IO8_FT 100MHz fast speed @ 1.2V"
io8_100m_ft_fs_pu_1v2  "IO8_FT 100MHz fast speed @ 1.2V pullup"
io8_100m_ft_fs_pd_1v2  "IO8_FT 100MHz fast speed @ 1.2V pulldown"
io8_100m_ft_ms_1v2  "IO8_FT 100MHz med speed @ 1.2V"
io8_100m_ft_ms_pu_1v2  "IO8_FT 100MHz med speed @ 1.2V pullup"
io8_100m_ft_ms_pd_1v2  "IO8_FT 100MHz med speed @ 1.2V pulldown"
io8_100m_ft_ls_1v2  "IO8_FT 100MHz low speed @ 1.2V"
io8_100m_ft_ls_pu_1v2  "IO8_FT 100MHz low speed @ 1.2V pullup"
io8_100m_ft_ls_pd_1v2  "IO8_FT 100MHz low speed @ 1.2V pulldown"
io8_100m_ft_hs_1v8  "IO8_FT 100MHz high speed @ 1.8V"
io8_100m_ft_hs_pu_1v8  "IO8_FT 100MHz high speed @ 1.8V pullup"
io8_100m_ft_hs_pd_1v8  "IO8_FT 100MHz high speed @ 1.8V pulldown"
io8_100m_ft_fs_1v8  "IO8_FT 100MHz fast speed @ 1.8V"
io8_100m_ft_fs_pu_1v8  "IO8_FT 100MHz fast speed @ 1.8V pullup"
io8_100m_ft_fs_pd_1v8  "IO8_FT 100MHz fast speed @ 1.8V pulldown"
io8_100m_ft_ms_1v8  "IO8_FT 100MHz med speed @ 1.8V"
io8_100m_ft_ms_pu_1v8  "IO8_FT 100MHz med speed @ 1.8V pullup"
io8_100m_ft_ms_pd_1v8  "IO8_FT 100MHz med speed @ 1.8V pulldown"
io8_100m_ft_ls_1v8  "IO8_FT 100MHz low speed @ 1.8V"
io8_100m_ft_ls_pu_1v8  "IO8_FT 100MHz low speed @ 1.8V pullup"
io8_100m_ft_ls_pd_1v8  "IO8_FT 100MHz low speed @ 1.8V pulldown"
io8_100m_ft_hs_3v3  "IO8_FT 100MHz high speed @ 3.3V"
io8_100m_ft_hs_pu_3v3  "IO8_FT 100MHz high speed @ 3.3V pullup"
io8_100m_ft_hs_pd_3v3  "IO8_FT 100MHz high speed @ 3.3V pulldown"
io8_100m_ft_fs_3v3  "IO8_FT 100MHz fast speed @ 3.3V"
io8_100m_ft_fs_pu_3v3  "IO8_FT 100MHz fast speed @ 3.3V pullup"
io8_100m_ft_fs_pd_3v3  "IO8_FT 100MHz fast speed @ 3.3V pulldown"
io8_100m_ft_ms_3v3  "IO8_FT 100MHz med speed @ 3.3V"
io8_100m_ft_ms_pu_3v3  "IO8_FT 100MHz med speed @ 3.3V pullup"
io8_100m_ft_ms_pd_3v3  "IO8_FT 100MHz med speed @ 3.3V pulldown"
io8_100m_ft_ls_3v3  "IO8_FT 100MHz low speed @ 3.3V"
io8_100m_ft_ls_pu_3v3  "IO8_FT 100MHz low speed @ 3.3V pullup"
io8_100m_ft_ls_pd_3v3  "IO8_FT 100MHz low speed @ 3.3V pulldown"
io8usb_id_nopu  "IOUSB ID @ 3.3V"
io8usb_id_pu  "IOUSB ID @ 3.3V pullup"
[Model Selector] io8_100m_usb_vbus_ft
io8_100m_ft_hs_1v2  "IO8_FT 100MHz high speed @ 1.2V"
io8_100m_ft_hs_pu_1v2  "IO8_FT 100MHz high speed @ 1.2V pullup"
io8_100m_ft_hs_pd_1v2  "IO8_FT 100MHz high speed @ 1.2V pulldown"
io8_100m_ft_fs_1v2  "IO8_FT 100MHz fast speed @ 1.2V"
io8_100m_ft_fs_pu_1v2  "IO8_FT 100MHz fast speed @ 1.2V pullup"
io8_100m_ft_fs_pd_1v2  "IO8_FT 100MHz fast speed @ 1.2V pulldown"
io8_100m_ft_ms_1v2  "IO8_FT 100MHz med speed @ 1.2V"
io8_100m_ft_ms_pu_1v2  "IO8_FT 100MHz med speed @ 1.2V pullup"
io8_100m_ft_ms_pd_1v2  "IO8_FT 100MHz med speed @ 1.2V pulldown"
io8_100m_ft_ls_1v2  "IO8_FT 100MHz low speed @ 1.2V"
io8_100m_ft_ls_pu_1v2  "IO8_FT 100MHz low speed @ 1.2V pullup"
io8_100m_ft_ls_pd_1v2  "IO8_FT 100MHz low speed @ 1.2V pulldown"
io8_100m_ft_hs_1v8  "IO8_FT 100MHz high speed @ 1.8V"
io8_100m_ft_hs_pu_1v8  "IO8_FT 100MHz high speed @ 1.8V pullup"
io8_100m_ft_hs_pd_1v8  "IO8_FT 100MHz high speed @ 1.8V pulldown"
io8_100m_ft_fs_1v8  "IO8_FT 100MHz fast speed @ 1.8V"
io8_100m_ft_fs_pu_1v8  "IO8_FT 100MHz fast speed @ 1.8V pullup"
io8_100m_ft_fs_pd_1v8  "IO8_FT 100MHz fast speed @ 1.8V pulldown"
io8_100m_ft_ms_1v8  "IO8_FT 100MHz med speed @ 1.8V"
io8_100m_ft_ms_pu_1v8  "IO8_FT 100MHz med speed @ 1.8V pullup"
io8_100m_ft_ms_pd_1v8  "IO8_FT 100MHz med speed @ 1.8V pulldown"
io8_100m_ft_ls_1v8  "IO8_FT 100MHz low speed @ 1.8V"
io8_100m_ft_ls_pu_1v8  "IO8_FT 100MHz low speed @ 1.8V pullup"
io8_100m_ft_ls_pd_1v8  "IO8_FT 100MHz low speed @ 1.8V pulldown"
io8_100m_ft_hs_3v3  "IO8_FT 100MHz high speed @ 3.3V"
io8_100m_ft_hs_pu_3v3  "IO8_FT 100MHz high speed @ 3.3V pullup"
io8_100m_ft_hs_pd_3v3  "IO8_FT 100MHz high speed @ 3.3V pulldown"
io8_100m_ft_fs_3v3  "IO8_FT 100MHz fast speed @ 3.3V"
io8_100m_ft_fs_pu_3v3  "IO8_FT 100MHz fast speed @ 3.3V pullup"
io8_100m_ft_fs_pd_3v3  "IO8_FT 100MHz fast speed @ 3.3V pulldown"
io8_100m_ft_ms_3v3  "IO8_FT 100MHz med speed @ 3.3V"
io8_100m_ft_ms_pu_3v3  "IO8_FT 100MHz med speed @ 3.3V pullup"
io8_100m_ft_ms_pd_3v3  "IO8_FT 100MHz med speed @ 3.3V pulldown"
io8_100m_ft_ls_3v3  "IO8_FT 100MHz low speed @ 3.3V"
io8_100m_ft_ls_pu_3v3  "IO8_FT 100MHz low speed @ 3.3V pullup"
io8_100m_ft_ls_pd_3v3  "IO8_FT 100MHz low speed @ 3.3V pulldown"
io8usb_adp "IOUSB ADP @ 3.3V"
io8usb_vbus "IOUSB VBUS @ 3.3V"
[Model Selector] io8_usb_ft
io8_100m_ft_hs_1v2  "IO8_FT 100MHz high speed @ 1.2V"
io8_100m_ft_hs_pu_1v2  "IO8_FT 100MHz high speed @ 1.2V pullup"
io8_100m_ft_hs_pd_1v2  "IO8_FT 100MHz high speed @ 1.2V pulldown"
io8_100m_ft_fs_1v2  "IO8_FT 100MHz fast speed @ 1.2V"
io8_100m_ft_fs_pu_1v2  "IO8_FT 100MHz fast speed @ 1.2V pullup"
io8_100m_ft_fs_pd_1v2  "IO8_FT 100MHz fast speed @ 1.2V pulldown"
io8_100m_ft_ms_1v2  "IO8_FT 100MHz med speed @ 1.2V"
io8_100m_ft_ms_pu_1v2  "IO8_FT 100MHz med speed @ 1.2V pullup"
io8_100m_ft_ms_pd_1v2  "IO8_FT 100MHz med speed @ 1.2V pulldown"
io8_100m_ft_ls_1v2  "IO8_FT 100MHz low speed @ 1.2V"
io8_100m_ft_ls_pu_1v2  "IO8_FT 100MHz low speed @ 1.2V pullup"
io8_100m_ft_ls_pd_1v2  "IO8_FT 100MHz low speed @ 1.2V pulldown"
io8_100m_ft_hs_1v8  "IO8_FT 100MHz high speed @ 1.8V"
io8_100m_ft_hs_pu_1v8  "IO8_FT 100MHz high speed @ 1.8V pullup"
io8_100m_ft_hs_pd_1v8  "IO8_FT 100MHz high speed @ 1.8V pulldown"
io8_100m_ft_fs_1v8  "IO8_FT 100MHz fast speed @ 1.8V"
io8_100m_ft_fs_pu_1v8  "IO8_FT 100MHz fast speed @ 1.8V pullup"
io8_100m_ft_fs_pd_1v8  "IO8_FT 100MHz fast speed @ 1.8V pulldown"
io8_100m_ft_ms_1v8  "IO8_FT 100MHz med speed @ 1.8V"
io8_100m_ft_ms_pu_1v8  "IO8_FT 100MHz med speed @ 1.8V pullup"
io8_100m_ft_ms_pd_1v8  "IO8_FT 100MHz med speed @ 1.8V pulldown"
io8_100m_ft_ls_1v8  "IO8_FT 100MHz low speed @ 1.8V"
io8_100m_ft_ls_pu_1v8  "IO8_FT 100MHz low speed @ 1.8V pullup"
io8_100m_ft_ls_pd_1v8  "IO8_FT 100MHz low speed @ 1.8V pulldown"
io8_100m_ft_hs_3v3  "IO8_FT 100MHz high speed @ 3.3V"
io8_100m_ft_hs_pu_3v3  "IO8_FT 100MHz high speed @ 3.3V pullup"
io8_100m_ft_hs_pd_3v3  "IO8_FT 100MHz high speed @ 3.3V pulldown"
io8_100m_ft_fs_3v3  "IO8_FT 100MHz fast speed @ 3.3V"
io8_100m_ft_fs_pu_3v3  "IO8_FT 100MHz fast speed @ 3.3V pullup"
io8_100m_ft_fs_pd_3v3  "IO8_FT 100MHz fast speed @ 3.3V pulldown"
io8_100m_ft_ms_3v3  "IO8_FT 100MHz med speed @ 3.3V"
io8_100m_ft_ms_pu_3v3  "IO8_FT 100MHz med speed @ 3.3V pullup"
io8_100m_ft_ms_pd_3v3  "IO8_FT 100MHz med speed @ 3.3V pulldown"
io8_100m_ft_ls_3v3  "IO8_FT 100MHz low speed @ 3.3V"
io8_100m_ft_ls_pu_3v3  "IO8_FT 100MHz low speed @ 3.3V pullup"
io8_100m_ft_ls_pd_3v3  "IO8_FT 100MHz low speed @ 3.3V pulldown"
io8_usb_fs_3v3  "IOUSB fast speed @ 3.3V"
io8_usb_fs_pu1_3v3  "IO8USB fast speed @ 3.3V pullup1"
io8_usb_fs_pd1_3v3  "IOUSB fast speed @ 3.3V pulldown1"
io8_usb_ls_3v3  "IOUSB low speed @ 3.3V"
io8_usb_ls_pu1_3v3  "IOUSB low speed @ 3.3V pullup1"
io8_usb_ls_pd1_3v3  "IOUSB low speed @ 3.3V pulldown1"
io8_usb_fs_pu2_3v3  "IOUSB fast speed @ 3.3V pullup2"
io8_usb_fs_pd2_3v3  "IOUSB fast speed @ 3.3V pulldown2"
io8_usb_ls_pu2_3v3  "IOUSB low speed @ 3.3V pullup2"
io8_usb_ls_pd2_3v3  "IOUSB low speed @ 3.3V pulldown2"
[Model Selector] io8_100m_i2c_ft
io8_100m_ft_hs_1v2  "IO8_FT 100MHz high speed @ 1.2V"
io8_100m_ft_hs_pu_1v2  "IO8_FT 100MHz high speed @ 1.2V pullup"
io8_100m_ft_hs_pd_1v2  "IO8_FT 100MHz high speed @ 1.2V pulldown"
io8_100m_ft_fs_1v2  "IO8_FT 100MHz fast speed @ 1.2V"
io8_100m_ft_fs_pu_1v2  "IO8_FT 100MHz fast speed @ 1.2V pullup"
io8_100m_ft_fs_pd_1v2  "IO8_FT 100MHz fast speed @ 1.2V pulldown"
io8_100m_ft_ms_1v2  "IO8_FT 100MHz med speed @ 1.2V"
io8_100m_ft_ms_pu_1v2  "IO8_FT 100MHz med speed @ 1.2V pullup"
io8_100m_ft_ms_pd_1v2  "IO8_FT 100MHz med speed @ 1.2V pulldown"
io8_100m_ft_ls_1v2  "IO8_FT 100MHz low speed @ 1.2V"
io8_100m_ft_ls_pu_1v2  "IO8_FT 100MHz low speed @ 1.2V pullup"
io8_100m_ft_ls_pd_1v2  "IO8_FT 100MHz low speed @ 1.2V pulldown"
io8_100m_ft_hs_1v8  "IO8_FT 100MHz high speed @ 1.8V"
io8_100m_ft_hs_pu_1v8  "IO8_FT 100MHz high speed @ 1.8V pullup"
io8_100m_ft_hs_pd_1v8  "IO8_FT 100MHz high speed @ 1.8V pulldown"
io8_100m_ft_fs_1v8  "IO8_FT 100MHz fast speed @ 1.8V"
io8_100m_ft_fs_pu_1v8  "IO8_FT 100MHz fast speed @ 1.8V pullup"
io8_100m_ft_fs_pd_1v8  "IO8_FT 100MHz fast speed @ 1.8V pulldown"
io8_100m_ft_ms_1v8  "IO8_FT 100MHz med speed @ 1.8V"
io8_100m_ft_ms_pu_1v8  "IO8_FT 100MHz med speed @ 1.8V pullup"
io8_100m_ft_ms_pd_1v8  "IO8_FT 100MHz med speed @ 1.8V pulldown"
io8_100m_ft_ls_1v8  "IO8_FT 100MHz low speed @ 1.8V"
io8_100m_ft_ls_pu_1v8  "IO8_FT 100MHz low speed @ 1.8V pullup"
io8_100m_ft_ls_pd_1v8  "IO8_FT 100MHz low speed @ 1.8V pulldown"
io8_100m_ft_hs_3v3  "IO8_FT 100MHz high speed @ 3.3V"
io8_100m_ft_hs_pu_3v3  "IO8_FT 100MHz high speed @ 3.3V pullup"
io8_100m_ft_hs_pd_3v3  "IO8_FT 100MHz high speed @ 3.3V pulldown"
io8_100m_ft_fs_3v3  "IO8_FT 100MHz fast speed @ 3.3V"
io8_100m_ft_fs_pu_3v3  "IO8_FT 100MHz fast speed @ 3.3V pullup"
io8_100m_ft_fs_pd_3v3  "IO8_FT 100MHz fast speed @ 3.3V pulldown"
io8_100m_ft_ms_3v3  "IO8_FT 100MHz med speed @ 3.3V"
io8_100m_ft_ms_pu_3v3  "IO8_FT 100MHz med speed @ 3.3V pullup"
io8_100m_ft_ms_pd_3v3  "IO8_FT 100MHz med speed @ 3.3V pulldown"
io8_100m_ft_ls_3v3  "IO8_FT 100MHz low speed @ 3.3V"
io8_100m_ft_ls_pu_3v3  "IO8_FT 100MHz low speed @ 3.3V pullup"
io8_100m_ft_ls_pd_3v3  "IO8_FT 100MHz low speed @ 3.3V pulldown"
io8_100m_i2c_ft_1v2  "IO8_FT 100MHz I2C @ 1.2V"
io8_100m_i2c_ft_pu_1v2  "IO8_FT 100MHz I2C @ 1.2V pullup"
io8_100m_i2c_ft_pd_1v2  "IO8_FT 100MHz I2C @ 1.2V pulldown"
io8_100m_i2c_ft_1v8  "IO8_FT 100MHz I2C @ 1.8V"
io8_100m_i2c_ft_pu_1v8  "IO8_FT 100MHz I2C @ 1.8V pullup"
io8_100m_i2c_ft_pd_1v8  "IO8_FT 100MHz I2C @ 1,8V pulldown"
io8_100m_i2c_ft_3v3  "IO8_FT 100MHz I2C @ 3.3V"
io8_100m_i2c_ft_pu_3v3  "IO8_FT 100MHz I2C HSLV @ 3.3V pullup"
io8_100m_i2c_ft_pd_3v3  "IO8_FT 100MHz I2C @ 3.3V pulldown"
[Model Selector] io8_166m_hslv_i2c_ft
io8_166m_ft_hs_1v2  "IO8_FT 166MHz high speed @ 1.2V"
io8_166m_ft_hs_pu_1v2  "IO8_FT 166MHz high speed @ 1.2V pullup"
io8_166m_ft_hs_pd_1v2  "IO8_FT 166MHz high speed @ 1.2V pulldown"
io8_166m_ft_fs_1v2  "IO8_FT 166MHz fast speed @ 1.2V"
io8_166m_ft_fs_pu_1v2  "IO8_FT 166MHz fast speed @ 1.2V pullup"
io8_166m_ft_fs_pd_1v2  "IO8_FT 166MHz fast speed @ 1.2V pulldown"
io8_166m_ft_ms_1v2  "IO8_FT 166MHz med speed @ 1.2V"
io8_166m_ft_ms_pu_1v2  "IO8_FT 166MHz med speed @ 1.2V pullup"
io8_166m_ft_ms_pd_1v2  "IO8_FT 166MHz med speed @ 1.2V pulldown"
io8_166m_ft_ls_1v2  "IO8_FT 166MHz low speed @ 1.2V"
io8_166m_ft_ls_pu_1v2  "IO8_FT 166MHz low speed @ 1.2V pullup"
io8_166m_ft_ls_pd_1v2  "IO8_FT 166MHz low speed @ 1.2V pulldown"
io8_166m_ft_hs_1v8  "IO8_FT 166MHz high speed @ 1.8V"
io8_166m_ft_hs_pu_1v8  "IO8_FT 166MHz high speed @ 1.8V pullup"
io8_166m_ft_hs_pd_1v8  "IO8_FT 166MHz high speed @ 1.8V pulldown"
io8_166m_ft_fs_1v8  "IO8_FT 166MHz fast speed @ 1.8V"
io8_166m_ft_fs_pu_1v8  "IO8_FT 166MHz fast speed @ 1.8V pullup"
io8_166m_ft_fs_pd_1v8  "IO8_FT 166MHz fast speed @ 1.8V pulldown"
io8_166m_ft_ms_1v8  "IO8_FT 166MHz med speed @ 1.8V"
io8_166m_ft_ms_pu_1v8  "IO8_FT 166MHz med speed @ 1.8V pullup"
io8_166m_ft_ms_pd_1v8  "IO8_FT 166MHz med speed @ 1.8V pulldown"
io8_166m_ft_ls_1v8  "IO8_FT 166MHz low speed @ 1.8V"
io8_166m_ft_ls_pu_1v8  "IO8_FT 166MHz low speed @ 1.8V pullup"
io8_166m_ft_ls_pd_1v8  "IO8_FT 166MHz low speed @ 1.8V pulldown"
io8_166m_ft_hs_3v3  "IO8_FT 166MHz high speed @ 3.3V"
io8_166m_ft_hs_pu_3v3  "IO8_FT 166MHz high speed @ 3.3V pullup"
io8_166m_ft_hs_pd_3v3  "IO8_FT 166MHz high speed @ 3.3V pulldown"
io8_166m_ft_fs_3v3  "IO8_FT 166MHz fast speed @ 3.3V"
io8_166m_ft_fs_pu_3v3  "IO8_FT 166MHz fast speed @ 3.3V pullup"
io8_166m_ft_fs_pd_3v3  "IO8_FT 166MHz fast speed @ 3.3V pulldown"
io8_166m_ft_ms_3v3  "IO8_FT 166MHz med speed @ 3.3V"
io8_166m_ft_ms_pu_3v3  "IO8_FT 166MHz med speed @ 3.3V pullup"
io8_166m_ft_ms_pd_3v3  "IO8_FT 166MHz med speed @ 3.3V pulldown"
io8_166m_ft_ls_3v3  "IO8_FT 166MHz low speed @ 3.3V"
io8_166m_ft_ls_pu_3v3  "IO8_FT 166MHz low speed @ 3.3V pullup"
io8_166m_ft_ls_pd_3v3  "IO8_FT 166MHz low speed @ 3.3V pulldown"
io8_166m_hslv_ft_hs_1v2  "IO8_FT 166MHz HSLV high speed @ 1.2V"
io8_166m_hslv_ft_hs_pu_1v2  "IO8_FT 166MHz HSLV high speed @ 1.2V pullup"
io8_166m_hslv_ft_hs_pd_1v2  "IO8_FT 166MHz HSLV high speed @ 1.2V pulldown"
io8_166m_hslv_ft_fs_1v2  "IO8_FT 166MHz HSLV fast speed @ 1.2V"
io8_166m_hslv_ft_fs_pu_1v2  "IO8_FT 166MHz HSLV fast speed @ 1.2V pullup"
io8_166m_hslv_ft_fs_pd_1v2  "IO8_FT 166MHz HSLV fast speed @ 1.2V pulldown"
io8_166m_hslv_ft_ms_1v2  "IO8_FT 166MHz HSLV med speed @ 1.2V"
io8_166m_hslv_ft_ms_pu_1v2  "IO8_FT 166MHz HSLV med speed @ 1.2V pullup"
io8_166m_hslv_ft_ms_pd_1v2  "IO8_FT 166MHz HSLV med speed @ 1.2V pulldown"
io8_166m_hslv_ft_ls_1v2  "IO8_FT 166MHz HSLV low speed @ 1.2V"
io8_166m_hslv_ft_ls_pu_1v2  "IO8_FT 166MHz HSLV low speed @ 1.2V pullup"
io8_166m_hslv_ft_ls_pd_1v2  "IO8_FT 166MHz HSLV low speed @ 1.2V pulldown"
io8_166m_hslv_ft_hs_1v8  "IO8_FT 166MHz HSLV high speed @ 1.8V"
io8_166m_hslv_ft_hs_pu_1v8  "IO8_FT 166MHz HSLV high speed @ 1.8V pullup"
io8_166m_hslv_ft_hs_pd_1v8  "IO8_FT 166MHz HSLV high speed @ 1.8V pulldown"
io8_166m_hslv_ft_fs_1v8  "IO8_FT 166MHz HSLV fast speed @ 1.8V"
io8_166m_hslv_ft_fs_pu_1v8  "IO8_FT 166MHz HSLV fast speed @ 1.8V pullup"
io8_166m_hslv_ft_fs_pd_1v8  "IO8_FT 166MHz HSLV fast speed @ 1.8V pulldown"
io8_166m_hslv_ft_ms_1v8  "IO8_FT 166MHz HSLV med speed @ 1.8V"
io8_166m_hslv_ft_ms_pu_1v8  "IO8_FT 166MHz HSLV med speed @ 1.8V pullup"
io8_166m_hslv_ft_ms_pd_1v8  "IO8_FT 166MHz HSLV med speed @ 1.8V pulldown"
io8_166m_hslv_ft_ls_1v8  "IO8_FT 166MHz HSLV low speed @ 1.8V"
io8_166m_hslv_ft_ls_pu_1v8  "IO8_FT 166MHz HSLV low speed @ 1.8V pullup"
io8_166m_hslv_ft_ls_pd_1v8  "IO8_FT 166MHz HSLV low speed @ 1.8V pulldown"
io8_166m_hslv_ft_hs_2v5  "IO8_FT 166MHz HSLV high speed @ 2.5V"
io8_166m_hslv_ft_hs_pu_2v5  "IO8_FT 166MHz HSLV high speed @ 2.5V pullup"
io8_166m_hslv_ft_hs_pd_2v5  "IO8_FT 166MHz HSLV high speed @ 2.5V pulldown"
io8_166m_hslv_ft_fs_2v5  "IO8_FT 166MHz HSLV fast speed @ 2.5V"
io8_166m_hslv_ft_fs_pu_2v5  "IO8_FT 166MHz HSLV fast speed @ 2.5V pullup"
io8_166m_hslv_ft_fs_pd_2v5  "IO8_FT 166MHz HSLV fast speed @ 2.5V pulldown"
io8_166m_hslv_ft_ms_2v5  "IO8_FT 166MHz HSLV med speed @ 2.5V"
io8_166m_hslv_ft_ms_pu_2v5  "IO8_FT 166MHz HSLV med speed @ 2.5V pullup"
io8_166m_hslv_ft_ms_pd_2v5  "IO8_FT 166MHz HSLV med speed @ 2.5V pulldown"
io8_166m_hslv_ft_ls_2v5  "IO8_FT 166MHz HSLV low speed @ 2.5V"
io8_166m_hslv_ft_ls_pu_2v5  "IO8_FT 166MHz HSLV low speed @ 2.5V pullup"
io8_166m_hslv_ft_ls_pd_2v5  "IO8_FT 166MHz HSLV low speed @ 2.5V pulldown"
io8_166m_i2c_ft_1v2  "IO8_FT 166MHz I2C @ 1.2V"
io8_166m_i2c_ft_pu_1v2  "IO8_FT 166MHz I2C @ 1.2V pullup"
io8_166m_i2c_ft_pd_1v2  "IO8_FT 166MHz I2C @ 1.2V pulldown"
io8_166m_i2c_ft_1v8  "IO8_FT 166MHz I2C @ 1.8V"
io8_166m_i2c_ft_pu_1v8  "IO8_FT 166MHz I2C @ 1.8V pullup"
io8_166m_i2c_ft_pd_1v8  "IO8_FT 166MHz I2C @ 1,8V pulldown"
io8_166m_i2c_ft_3v3  "IO8_FT 166MHz I2C @ 3.3V"
io8_166m_i2c_ft_pu_3v3  "IO8_FT 166MHz I2C HSLV @ 3.3V pullup"
io8_166m_i2c_ft_pd_3v3  "IO8_FT 166MHz I2C @ 3.3V pulldown"
| Models and submodels in the file (212): io8_100m_ft_hs_1v2 (I/O), io8_100m_ft_hs_pu_1v2 (I/O), io8_100m_ft_hs_pd_1v2 (I/O), io8_100m_ft_fs_1v2 (I/O), io8_100m_ft_fs_pu_1v2 (I/O), io8_100m_ft_fs_pd_1v2 (I/O), io8_100m_ft_ms_1v2 (I/O), io8_100m_ft_ms_pu_1v2 (I/O), io8_100m_ft_ms_pd_1v2 (I/O), io8_100m_ft_ls_1v2 (I/O), io8_100m_ft_ls_pu_1v2 (I/O), io8_100m_ft_ls_pd_1v2 (I/O), io8_100m_ft_hs_1v8 (I/O), io8_100m_ft_hs_pu_1v8 (I/O), io8_100m_ft_hs_pd_1v8 (I/O), io8_100m_ft_fs_1v8 (I/O), io8_100m_ft_fs_pu_1v8 (I/O), io8_100m_ft_fs_pd_1v8 (I/O), io8_100m_ft_ms_1v8 (I/O), io8_100m_ft_ms_pu_1v8 (I/O), io8_100m_ft_ms_pd_1v8 (I/O), io8_100m_ft_ls_1v8 (I/O), io8_100m_ft_ls_pu_1v8 (I/O), io8_100m_ft_ls_pd_1v8 (I/O), io8_100m_ft_hs_3v3 (I/O), io8_100m_ft_hs_pu_3v3 (I/O), io8_100m_ft_hs_pd_3v3 (I/O), io8_100m_ft_fs_3v3 (I/O), io8_100m_ft_fs_pu_3v3 (I/O), io8_100m_ft_fs_pd_3v3 (I/O), io8_100m_ft_ms_3v3 (I/O), io8_100m_ft_ms_pu_3v3 (I/O), io8_100m_ft_ms_pd_3v3 (I/O), io8_100m_ft_ls_3v3 (I/O), io8_100m_ft_ls_pu_3v3 (I/O), io8_100m_ft_ls_pd_3v3 (I/O), io8_100m_hslv_ft_hs_1v2 (I/O), io8_100m_hslv_ft_hs_pu_1v2 (I/O), io8_100m_hslv_ft_hs_pd_1v2 (I/O), io8_100m_hslv_ft_fs_1v2 (I/O), io8_100m_hslv_ft_fs_pu_1v2 (I/O), io8_100m_hslv_ft_fs_pd_1v2 (I/O), io8_100m_hslv_ft_ms_1v2 (I/O), io8_100m_hslv_ft_ms_pu_1v2 (I/O), io8_100m_hslv_ft_ms_pd_1v2 (I/O), io8_100m_hslv_ft_ls_1v2 (I/O), io8_100m_hslv_ft_ls_pu_1v2 (I/O), io8_100m_hslv_ft_ls_pd_1v2 (I/O), io8_100m_hslv_ft_hs_1v8 (I/O), io8_100m_hslv_ft_hs_pu_1v8 (I/O), io8_100m_hslv_ft_hs_pd_1v8 (I/O), io8_100m_hslv_ft_fs_1v8 (I/O), io8_100m_hslv_ft_fs_pu_1v8 (I/O), io8_100m_hslv_ft_fs_pd_1v8 (I/O), io8_100m_hslv_ft_ms_1v8 (I/O), io8_100m_hslv_ft_ms_pu_1v8 (I/O), io8_100m_hslv_ft_ms_pd_1v8 (I/O), io8_100m_hslv_ft_ls_1v8 (I/O), io8_100m_hslv_ft_ls_pu_1v8 (I/O), io8_100m_hslv_ft_ls_pd_1v8 (I/O), io8_100m_hslv_ft_hs_2v5 (I/O), io8_100m_hslv_ft_hs_pu_2v5 (I/O), io8_100m_hslv_ft_hs_pd_2v5 (I/O), io8_100m_hslv_ft_fs_2v5 (I/O), io8_100m_hslv_ft_fs_pu_2v5 (I/O), io8_100m_hslv_ft_fs_pd_2v5 (I/O), io8_100m_hslv_ft_ms_2v5 (I/O), io8_100m_hslv_ft_ms_pu_2v5 (I/O), io8_100m_hslv_ft_ms_pd_2v5 (I/O), io8_100m_hslv_ft_ls_2v5 (I/O), io8_100m_hslv_ft_ls_pu_2v5 (I/O), io8_100m_hslv_ft_ls_pd_2v5 (I/O), io8_166m_ft_hs_1v2 (I/O), io8_166m_ft_hs_pu_1v2 (I/O), io8_166m_ft_hs_pd_1v2 (I/O), io8_166m_ft_fs_1v2 (I/O), io8_166m_ft_fs_pu_1v2 (I/O), io8_166m_ft_fs_pd_1v2 (I/O), io8_166m_ft_ms_1v2 (I/O), io8_166m_ft_ms_pu_1v2 (I/O)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
